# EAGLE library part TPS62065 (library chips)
Step down DC-DC converter.
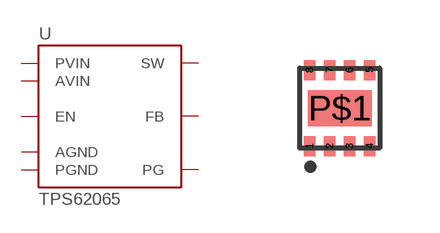
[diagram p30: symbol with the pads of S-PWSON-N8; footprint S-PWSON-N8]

Designator prefix U

## TPS62065 (DIGIKEY: 296-39441-1-ND)  [S-PWSON-N8]
1  PGND
2  SW
3  AGND
4  FB
5  EN
6  PG
7  AVIN
8  PVIN
P$1  PGND

## Footprint S-PWSON-N8 (pad centres in mm)
smd 0.28 x 0.5: 1 -0.75,-0.95; 2 -0.25,-0.95; 3 0.25,-0.95; 4 0.75,-0.95; 5 0.75,0.95; 6 0.25,0.95; 7 -0.25,0.95; 8 -0.75,0.95
smd 1.6 x 0.9: P$1 0,0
